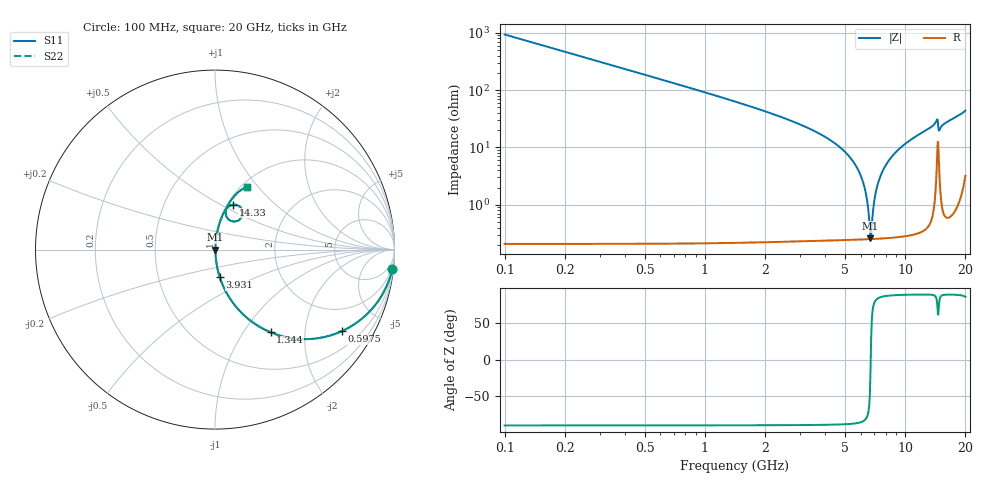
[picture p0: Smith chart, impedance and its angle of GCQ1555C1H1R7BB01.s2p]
!Murata Part Number: GCQ1555C1H1R7BB01
!These Parameters are Measured in Series Mode Connection
!Data Generated on Mar 13, 2026
!  o--ll--o
!Port1  Port2
!  o------o
!Operation Temp=25[degC], DC Bias Voltage=0[V]
!Freq. Start=100[MHz] Stop=20[GHz] 401[Steps]
# Hz S RI R 50
!Freq.(Hz) S11(Real) S11(Imag) S21(Real) S21(Imag) S12(Real) S12(Imag) S22(Real) S22(Imag)
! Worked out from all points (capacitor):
!   401 points, 100 MHz to 20 GHz, reference 50 ohm
!   read as one part in series: C = 1.7 pF near 199.5 MHz
!   lowest |Z| = 262 mohm at 6.717 GHz (marker M1)
!   series resonance near 6.734 GHz, so ESL is about 330 pH
!   S11 on the Smith chart (normalised r, x): 100 MHz: 1, -19; 597.5 MHz: 1.00, -3.11; 1.344 GHz: 1.00, -1.34; 3.931 GHz: 1.00, -0.31; 14.33 GHz: 1.06, +0.58; 20 GHz: 1.06, +0.88
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1e8  0.9887 -0.1056  0.0113 0.1056  0.0113 0.1056  0.9887 -0.1056
3.4875e8  0.8774 -0.3276  0.1226 0.3276  0.1226 0.3276  0.8774 -0.3276
5.975e8  0.7071 -0.4544  0.2929 0.4544  0.2929 0.4544  0.7071 -0.4544
1.34375e9  0.3098 -0.4608  0.6902 0.4608  0.6902 0.4608  0.3098 -0.4608
2.13975e9  0.1355 -0.3394  0.8645 0.3394  0.8645 0.3394  0.1355 -0.3394
3.43325e9  0.0413 -0.1933  0.9587 0.1933  0.9587 0.1933  0.0413 -0.1933
3.93075e9  0.0263 -0.1528  0.9737 0.1528  0.9737 0.1528  0.0263 -0.1528
5.12475e9  0.0083 -0.0764  0.9917 0.0764  0.9917 0.0764  0.0083 -0.0764
5.92075e9  0.00376 -0.0359  0.9962 0.0359  0.9962 0.0359  0.00376 -0.0359
6.3685e9  0.00273 -0.0155  0.9973 0.0155  0.9973 0.0155  0.00273 -0.0155
6.71675e9  0.00251 -0.000715  0.9975 0.000715  0.9975 0.000715  0.00251 -0.000715
6.7665e9  0.00252 0.00134  0.9975 -0.00134  0.9975 -0.00134  0.00252 0.00134
6.9655e9  0.00262 0.00943  0.9974 -0.00943  0.9974 -0.00943  0.00262 0.00943
7.11475e9  0.00277 0.0154  0.9972 -0.0154  0.9972 -0.0154  0.00277 0.0154
7.662e9  0.00389 0.0361  0.9961 -0.0361  0.9961 -0.0361  0.00389 0.0361
8.60725e9  0.00748 0.0692  0.9925 -0.0692  0.9925 -0.0692  0.00748 0.0692
1.005e10  0.0162 0.1147  0.9838 -0.1147  0.9838 -0.1147  0.0162 0.1147
1.338325e10  0.0517 0.2109  0.9483 -0.2109  0.9483 -0.2109  0.0517 0.2109
1.43285e10  0.1012 0.2506  0.8988 -0.2506  0.8988 -0.2506  0.1012 0.2506
1.477625e10  0.0754 0.1683  0.9246 -0.1683  0.9246 -0.1683  0.0754 0.1683
1.67165e10  0.0855 0.2696  0.9145 -0.2696  0.9145 -0.2696  0.0855 0.2696
2e10  0.179 0.3485  0.821 -0.3485  0.821 -0.3485  0.179 0.3485
